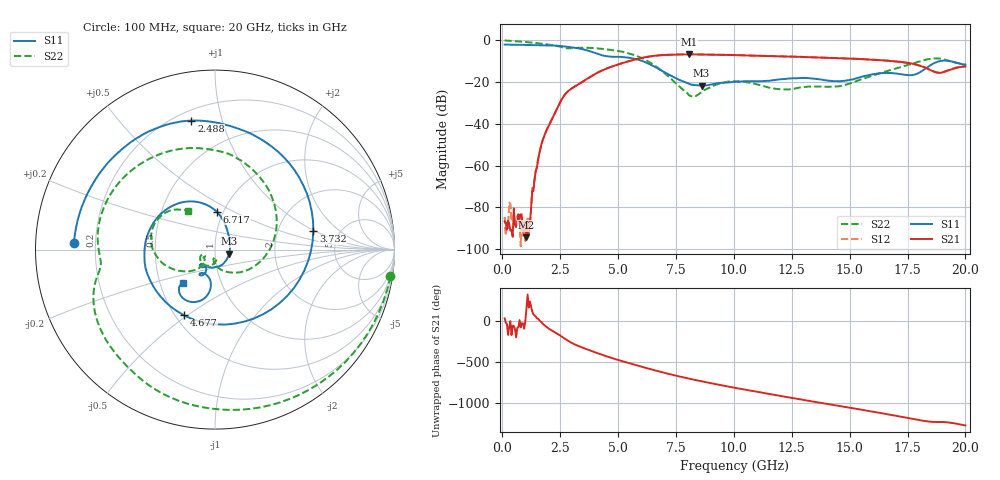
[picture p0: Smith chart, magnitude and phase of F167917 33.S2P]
!  2-Port S-parameters saved by WinCal
! VAR MeasName=S-Parameters (CALIBRATED_DATA) read from VNA (N5242A)
! VAR MeasDate=2016-11-22 9:01:23
! VAR NAME=F167917 33
! VAR FILENAME=F167917 33.S2P
! VAR DATE=2016-11-22 9:01:23
! VAR PHYS_PORTS=1,2
# Hz S DB R 50
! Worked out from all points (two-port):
!   401 points, 100 MHz to 20 GHz, reference 50 ohm
!   highest |S21| = -6.73 dB at 8.06 GHz (marker M1); lowest = -94.3 dB at 1.045 GHz (marker M2)
!   |S21| within 3 dB of the highest: 5.571 GHz to 16.54 GHz (10.97 GHz wide, 99.2 % of centre)
!   lowest |S11| = -21.8 dB at 8.607 GHz (marker M3), VSWR 1.18, Z = 58.5 - j2.59 ohm
!   |S11| at or under -10 dB: 6.053 GHz to 18.9 GHz (12.85 GHz wide, 103 % of centre); 19.34 GHz to end of sweep
!   |S22| runs from -26.9 to -0.1 dB; largest |S21 - S12| = 0.005
!   S11 on the Smith chart (normalised r, x): 100 MHz: 0.12, +0.02; 2.488 GHz: 0.26, +0.80; 3.732 GHz: 3.21, +0.95; 4.677 GHz: 0.55, -0.49; 6.717 GHz: 0.93, +0.41; 20 GHz: 0.66, -0.26
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1e8  -2.09 177.3  -86.81 32.1  -84.63 40.7  -0.10 -8.7
1.04525e9  -2.23 151.9  -94.34 163.2  -93.04 -12.6  -0.88 -80.9
1.24425e9  -2.26 146.2  -80.56 172.8  -80.46 150.5  -1.09 -94.0
1.74175e9  -2.37 130.7  -47.94 -33.1  -47.99 -32.9  -1.72 -124.2
2.488e9  -2.73 100.3  -29.89 -176.8  -29.90 -177.3  -3.08 -163.3
3.43325e9  -4.19 40.5  -20.10 37.2  -20.13 37.2  -3.57 164.6
3.73175e9  -5.08 10.6  -17.98 5.2  -17.99 5.5  -3.63 151.3
4.22925e9  -6.96 -53.6  -14.88 -45.8  -14.84 -45.6  -4.04 128.3
4.677e9  -7.85 -115.3  -12.84 -88.3  -12.77 -88.4  -4.62 106.4
5.1745e9  -8.00 -170.3  -10.96 -130.6  -10.91 -130.9  -5.48 79.1
5.7715e9  -9.03 141.7  -9.13 -179.3  -9.14 -179.7  -7.39 41.2
6.71675e9  -13.49 87.2  -7.25 107.0  -7.29 107.0  -13.18 -30.3
6.7665e9  -13.81 85.1  -7.20 103.4  -7.24 103.2  -13.61 -34.2
8.06e9  -20.80 25.2  -6.73 16.0  -6.74 16.0  -26.38 -98.3
8.60725e9  -21.77 -15.7  -6.84 -17.2  -6.84 -17.2  -24.82 -82.5
1.005e10  -19.77 -100.4  -7.10 -97.1  -7.10 -97.0  -19.72 -131.4
1.1642e10  -19.23 -120.6  -7.60 -177.7  -7.57 -177.7  -22.96 -157.7
1.338325e10  -18.33 -134.3  -8.16 97.8  -8.14 97.9  -22.14 -145.9
1.51245e10  -18.76 -115.3  -8.82 15.3  -8.79 15.1  -20.26 -129.0
1.67165e10  -15.66 -121.1  -9.82 -63.0  -9.84 -63.1  -14.44 -140.4
1.85075e10  -11.85 -99.3  -14.38 -150.6  -14.29 -150.7  -8.86 171.7
2e10  -11.77 -133.3  -12.54 164.3  -12.44 164.0  -11.59 124.3
